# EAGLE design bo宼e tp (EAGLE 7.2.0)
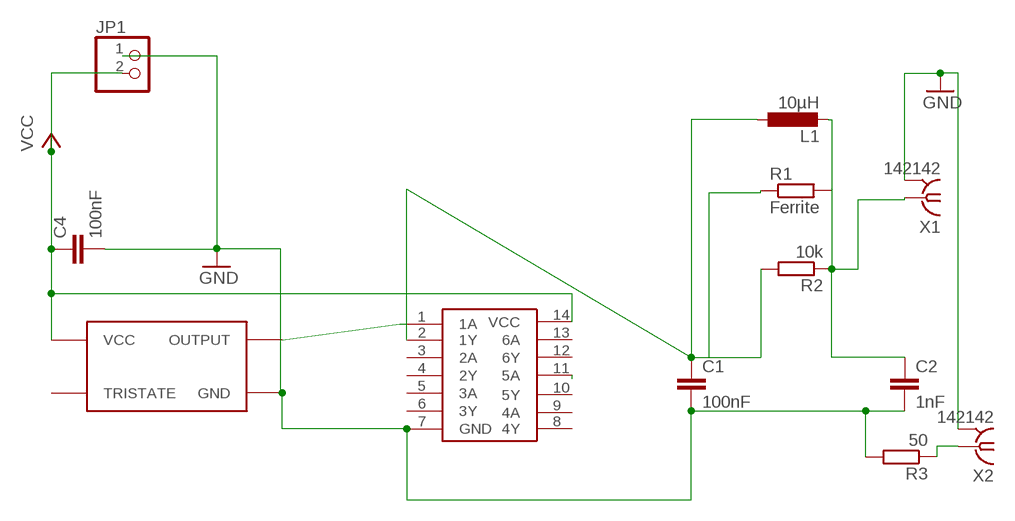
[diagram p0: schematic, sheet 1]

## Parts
C1  100nF  C-EU025-025X050  [C025-025X050]
C2  1nF  C-EU025-025X050  [C025-025X050]
C4  100nF  C-EU025-025X050  [C025-025X050]
JP1  PINHD-1X2  [1X02]
L1  10µH  L-EU0204/5  [0204/5]
O1  OSCILLATEUR16MHZ  [OSCILLATEUR16MHZ]
R1  Ferrite  R-EU_0204/2V  [0204V]
R2  10k  R-EU_0204/2V  [0204V]
R3  50  R-EU_0204/2V  [0204V]
U$1  CD74AC14E  [CD74AC14E]
X1  142142  [142142]
X2  142142  [142142]

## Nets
GND: C4.2 JP1.1 X1.2 X1.3 X1.4 X1.5 X2.2 X2.3 X2.4 X2.5
N$3: C1.2 C2.2 O1.GND R3.2 U$1.7(GND)
N$10: C2.1 L1.2 R1.2 R2.1 X1.1
N$11: C1.1 L1.1 R1.1 R2.2 U$1.2(1Y)
N$12: U$1.11(5A)
N$18: R3.1 X2.1
OUTPUT_16MHZ: O1.OUTPUT U$1.1(1A)
VCC: C4.1 JP1.2 O1.VCC U$1.14(VCC)
Unconnected: O1.P$1(TRISTATE) U$1.3(2A) U$1.4(2Y) U$1.5(3A) U$1.6(3Y) U$1.8(4Y) U$1.9(4A) U$1.10(5Y) U$1.12(6Y) U$1.13(6A)

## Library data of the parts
C1 C2 C4 = resistor:C-EU: CAPACITOR, European symbol
JP1 = pinhead:PINHD-1X2: PIN HEADER
L1 = resistor:L-EU: INDUCTOR, European symbol
O1 = Oscillateur 16MHz:OSCILLATEUR16MHZ
R1-R3 = resistor:R-EU_: RESISTOR, European symbol
U$1 = CD74AC14E:CD74AC14E
X1 X2 = BNC-female:142142: Amphenol Connex 142142; MF: Amphenol Connex; MPN: 142142; OC_FARNELL: unknown; OC_NEWARK: unknown

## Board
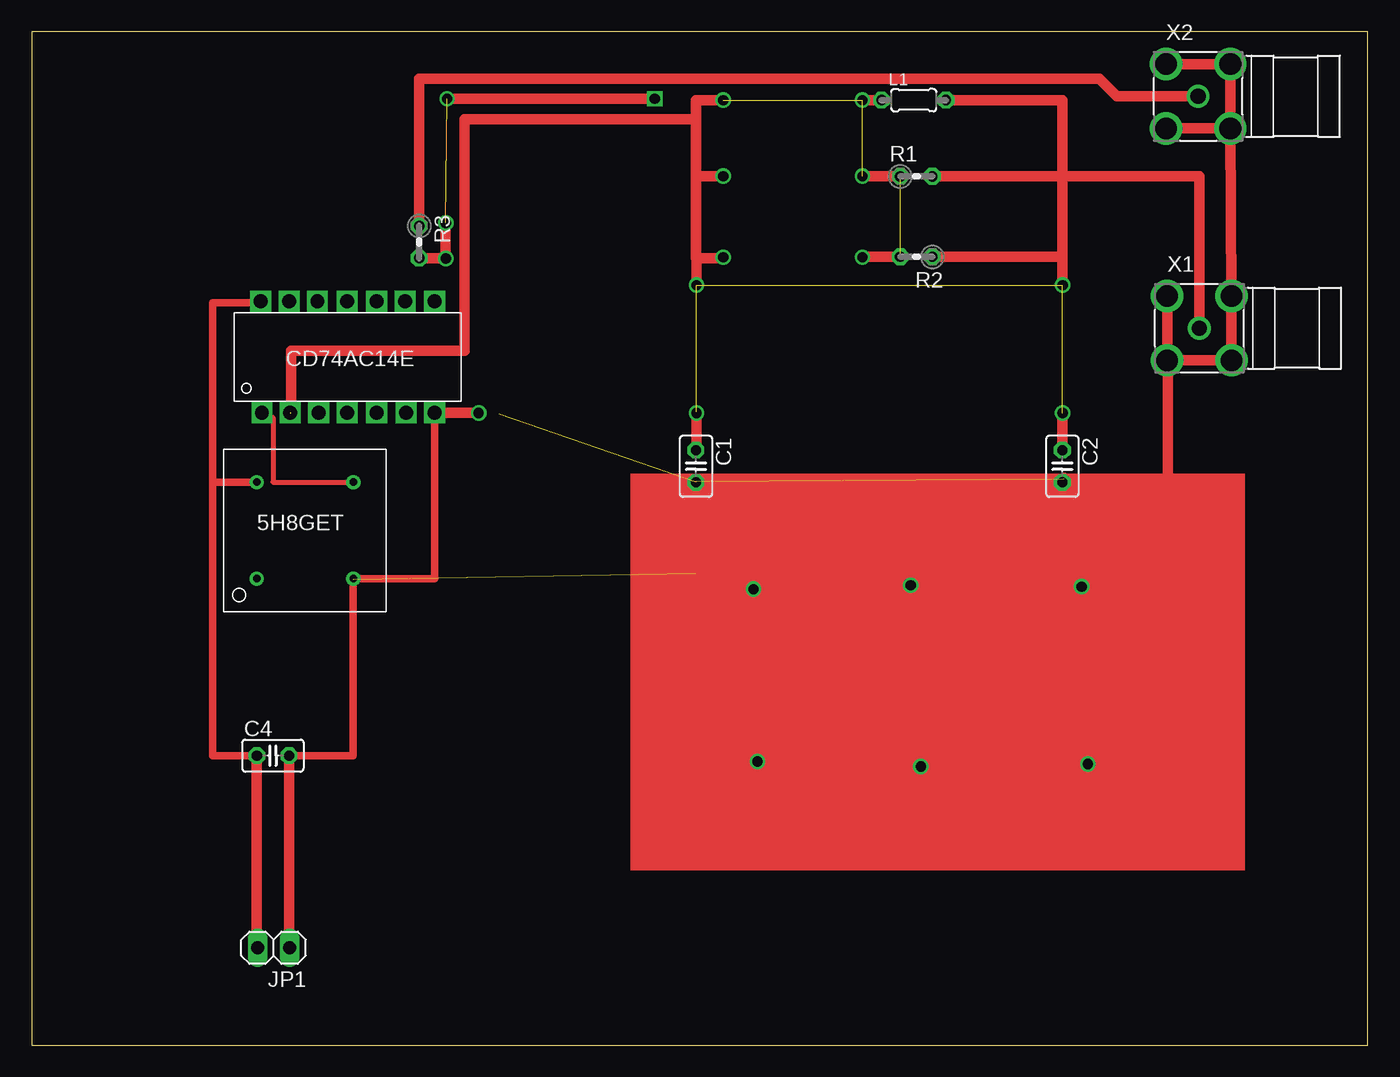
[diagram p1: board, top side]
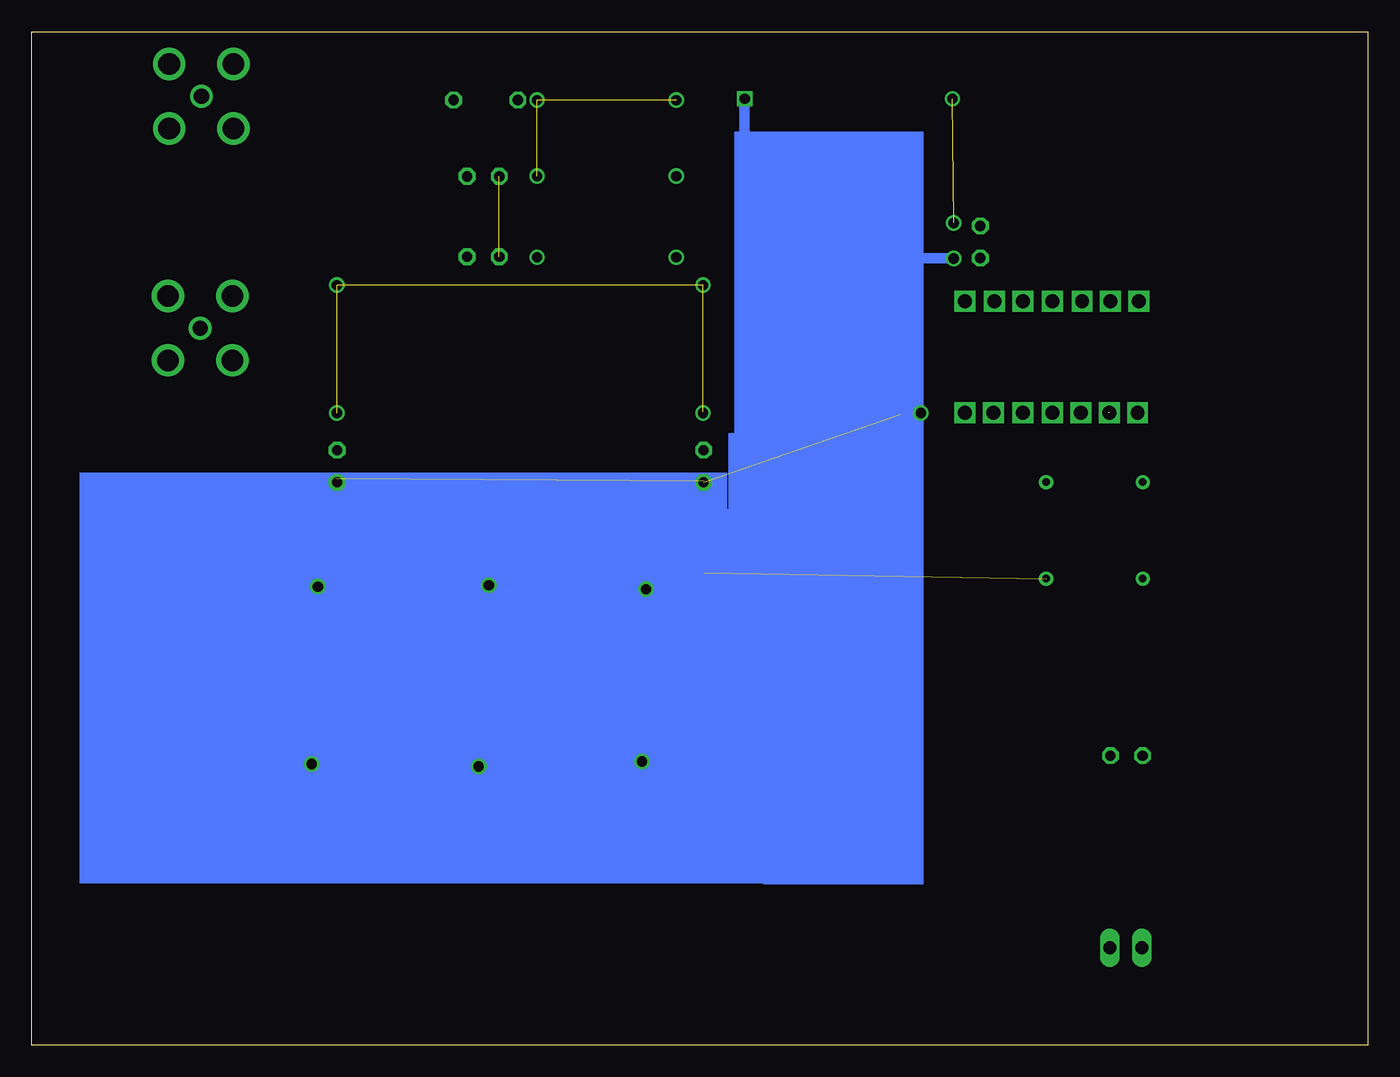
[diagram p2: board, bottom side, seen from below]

Size 105.5 x 80 mm. Coordinates in mm from the lower left corner, seen from the top.
Outline: 0,0 105.5,0 105.5,80 0,80 0,0
Copper layers (1*16): Top 0.035mm / dielectric 1.5mm / Bottom 0.035mm
Design rules "default": minimum track width 10mil, minimum drill 24mil, track to track 8mil, track to pad 8mil, pad to pad 8mil, via to via 8mil, smd to smd 8mil, copper to edge 40mil, drill to drill 8mil, minimum pad ring 10mil, minimum via ring 8mil, stop-mask expansion 4mil, vias tented up to drill 0mil, thermal gap 10mil

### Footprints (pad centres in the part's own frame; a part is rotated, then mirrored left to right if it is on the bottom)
C025-025X050 = drill 0.8 octagon: 1 -1.27,0; 2 1.27,0
1X02 = drill 1.016 long: 1 -1.27,0; 2 1.27,0
0204/5 = drill 0.813 octagon: 1 -2.54,0; 2 2.54,0
OSCILLATEUR16MHZ = drill 0.6: GND 7.62,0; OUTPUT 7.62,7.62; P$1 0,0; VCC 0,7.62
0204V = drill 0.813 octagon: 1 -1.27,0; 2 1.27,0
CD74AC14E = drill 1.1 square: 1 -7.22,0.4; 2 -4.98,0.4; 3 -2.74,0.4; 4 -0.5,0.4; 5 1.84,0.4; 6 4.18,0.4; 7 6.42,0.4; 8 6.42,9.19; 9 4.08,9.19; 10 1.84,9.19; 11 -0.5,9.19; 12 -2.84,9.19; 13 -5.08,9.19; 14 -7.32,9.19
142142 = drill 1.2: 1 0,0 | drill 1.7: 2 -2.54,2.54; 3 2.54,2.54; 4 2.54,-2.54; 5 -2.54,-2.54

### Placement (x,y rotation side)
C1  52.45,45.7 270 top
C2  81.38,45.7 270 top
C4  19.05,22.86 0 top
JP1  19.1,7.7 180 top
L1  69.65,74.6 0 top
O1  17.78,36.83 0 top
R1  69.85,68.58 0 top
R2  69.85,62.23 180 top
R3  30.6,63.4 270 top
U$1  25.4,49.53 0 top
X1  92.2,56.6 0 top
X2  92.1,74.9 0 top

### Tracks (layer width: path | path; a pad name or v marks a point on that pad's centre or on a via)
GND  (2 unrouted)
  Top 0.61: C4.2 25.4,22.86 25.4,36.8
  Top 0.813: JP1.1 20.32,7.7 C4.2 | 52.4,37.24 52.4,44.5 | X2.4 X2.3 X2.2 | X2.4 X2.5 | X2.4 X1.3 X1.4 X1.5 | X1.2 X1.5 | X1.5 89.7,54.06 89.7,44.7 81.5,44.7 81.5,44.8
N$1  (via drill 0.8)
  other vias: 57,36
N$2  (via drill 0.8)
  other vias: 57.3,22.4
N$3  (via drill 0.8)  (2 unrouted)
  Top 0.61: O1.GND 31.82,36.83 U$1.7
  Top 0.813: U$1.7 35.3,49.93 v35.3,49.9 | R3.2 32.7,62.13 | 32.7,62.13 v32.7,62.1 | 32.8,64.9 v32.7,64.9 32.7,62.13 | 32.8,74.7 v49.2,74.7 | C1.2 81.38,44.53 C2.2
  Bottom 0.813: v35.3,49.9 36.9,49.9 | 36.9,49.9 36.9,49.8 | v32.7,62.1 36.9,62.1 36.9,49.9 | v49.2,74.7 49.2,70.5
N$8  (via drill 0.8)
  other vias: 70.2,22
N$9  (via drill 0.8)
  other vias: 83.4,22.2
N$10  (1 unrouted)
  Top 0.406: R1.2 81.4,68.58 81.4,68.8
  Top 0.813: C2.1 81.38,49.88 81.4,49.9 | R2.1 81.4,62.23 | 81.4,62.23 81.4,60 | L1.2 81.4,74.6 81.4,68.8 81.4,62.23 | R1.2 92.2,68.58 X1.1
N$11  (5 unrouted)
  Top 0.813: R2.2 65.6,62.23 65.6,62.2 | R1.1 65.6,68.58 65.6,68.6 | 54.6,62.2 54.6,62.1 52.5,62.1 | 52.5,62.1 52.45,62.1 52.45,68.6 | 52.45,73.1 52.45,74.6 54.6,74.6 | 52.45,73.1 52.45,68.6 | 52.45,68.6 54.6,68.6 | L1.1 65.6,74.6 | C1.1 52.5,47.07 52.5,50 | 20.5,49.93 20.5,54.8 34.2,54.8 34.2,73.1 52.45,73.1 | 52.5,60 52.5,62.1
N$13  (via drill 0.8)
  other vias: 32.8,74.7
N$15  (via drill 0.8)
  other vias: 54.6,68.6
N$17  (via drill 0.8)
  other vias: 54.6,62.2
N$18
  Top 0.813: X2.1 85.7,74.9 84.3,76.3 30.6,76.3 R3.1
N$19  (via drill 0.8)
  other vias: 82.9,36.2
N$21  (via drill 0.8)
  other vias: 65.6,74.6
N$22  (via drill 0.8)
  other vias: 69.4,36.3
N$23  (via drill 0.8)
  other vias: 65.6,68.6
N$24  (via drill 0.8)
  other vias: 65.6,62.2
N$25  (via drill 0.8)
  other vias: 54.6,74.6
N$26  (via drill 0.8)
  other vias: 52.5,49.9
N$27  (via drill 0.8)  (1 unrouted)
  other vias: 52.5,60 81.4,60
N$29  (via drill 0.8)
  other vias: 81.4,49.9
N$30  (via drill 0.8)
  other vias: 32.7,62.1
OUTPUT_16MHZ
  Top 0.406: U$1.1 19.05,49.53 19.05,44.45 O1.OUTPUT
VCC
  Top 0.61: O1.VCC 14.3,44.45 | 14.3,44.45 14.3,58.6 18.08,58.6 U$1.14 | C4.1 14.3,22.86 14.3,44.45
  Top 0.813: JP1.2 17.78,7.7 C4.1
(copper drawn outside any net)
  shapes: Bottom area x7, Top area x1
